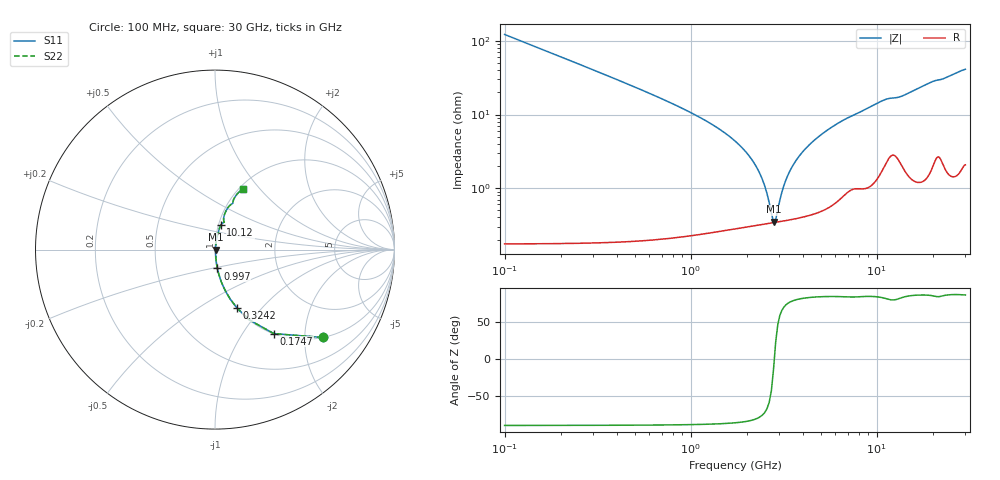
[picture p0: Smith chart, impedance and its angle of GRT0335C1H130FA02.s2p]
!Murata Part Number: GRT0335C1H130FA02
!These Parameters are Measured in Series Mode Connection
!Data Generated on Jun 19, 2026
!  o--ll--o
!Port1  Port2
!  o------o
!Operation Temp=25[degC], DC Bias Voltage=0[V]
!Freq. Start=100[MHz] Stop=30[GHz] 401[Steps]
# Hz S RI R 50
!Freq.(Hz) S11(Real) S11(Imag) S21(Real) S21(Imag) S12(Real) S12(Imag) S22(Real) S22(Imag)
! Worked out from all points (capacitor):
!   401 points, 100 MHz to 30 GHz, reference 50 ohm
!   read as one part in series: C = 13 pF near 249.5 MHz
!   lowest |Z| = 349 mohm at 2.791 GHz (marker M1)
!   series resonance near 2.818 GHz, so ESL is about 250 pH
!   S11 on the Smith chart (normalised r, x): 100 MHz: 1.00, -2.45; 174.8 MHz: 1.00, -1.40; 324.2 MHz: 1.00, -0.74; 997 MHz: 1.00, -0.21; 10.12 GHz: 1.03, +0.29; 30 GHz: 1.04, +0.82
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1e8  0.599 -0.4894  0.401 0.4894  0.401 0.4894  0.599 -0.4894
1.7475e8  0.3279 -0.4682  0.6721 0.4682  0.6721 0.4682  0.3279 -0.4682
3.2425e8  0.123 -0.326  0.877 0.326  0.877 0.326  0.123 -0.326
5.485e8  0.0456 -0.2042  0.9544 0.2042  0.9544 0.2042  0.0456 -0.2042
9.97e8  0.0135 -0.1053  0.9865 0.1053  0.9865 0.1053  0.0135 -0.1053
1.7445e9  0.00462 -0.0426  0.9954 0.0426  0.9954 0.0426  0.00462 -0.0426
2.11825e9  0.00364 -0.0247  0.9964 0.0247  0.9964 0.0247  0.00364 -0.0247
2.41725e9  0.00336 -0.0131  0.9966 0.0131  0.9966 0.0131  0.00336 -0.0131
2.71625e9  0.00336 -0.00312  0.9966 0.00312  0.9966 0.00312  0.00336 -0.00312
2.791e9  0.00338 -0.000803  0.9966 0.000803  0.9966 0.000803  0.00338 -0.000803
2.9405e9  0.00347 0.00366  0.9965 -0.00366  0.9965 -0.00366  0.00347 0.00366
3.16475e9  0.00367 0.00995  0.9963 -0.00995  0.9963 -0.00995  0.00367 0.00995
3.31425e9  0.00384 0.0139  0.9962 -0.0139  0.9962 -0.0139  0.00384 0.0139
3.688e9  0.00438 0.0233  0.9956 -0.0233  0.9956 -0.0233  0.00438 0.0233
4.286e9  0.00557 0.0369  0.9944 -0.0369  0.9944 -0.0369  0.00557 0.0369
5.10825e9  0.00782 0.0539  0.9922 -0.0539  0.9922 -0.0539  0.00782 0.0539
6.8275e9  0.0156 0.0849  0.9844 -0.0849  0.9844 -0.0849  0.0156 0.0849
1.01165e10  0.0325 0.1361  0.9675 -0.1361  0.9675 -0.1361  0.0325 0.1361
1.505e10  0.0502 0.186  0.9498 -0.186  0.9498 -0.186  0.0502 0.186
2.005825e10  0.0886 0.2511  0.9114 -0.2511  0.9114 -0.2511  0.0886 0.2511
2.50665e10  0.114 0.2972  0.886 -0.2972  0.886 -0.2972  0.114 0.2972
3e10  0.1574 0.3398  0.8426 -0.3398  0.8426 -0.3398  0.1574 0.3398
